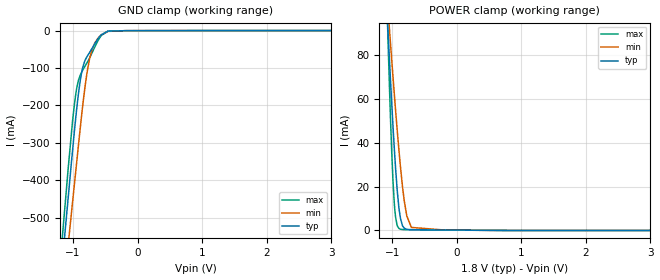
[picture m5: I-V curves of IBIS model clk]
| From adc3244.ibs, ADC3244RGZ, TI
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|   clk Model
[Model]   clk
Model_type   Input
Vinl = 0.4
Vinh = 1.2
|   typ   min   max
|   (nom PVT)   (fast PVT)   (slow PVT)
C_comp   2.914e-12   2.780e-12   2.974e-12
| Where nom  PVT is Nominal Process, 1.8V, 27C
|   Fast PVT is Strong Process,  1.9V, -40C
|   Slow PVT is Weak Process,   1.7V, 125C
[Voltage Range]   1.8   1.7   1.9
|Junction Temperature
[Temperature Range]   27   125   -40
[Power Clamp Reference]   1.8   1.7   1.9
[GND Clamp Reference]   0   0   0
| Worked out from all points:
|   POWER clamp passes 1 mA (typ) near -0.81 V on its own axis
[GND Clamp]
|   Voltage   I(typ)   I(min)   I(max)
-1.8V     -1.823A    -1.811A    -1.849A
-1.373V   -1.008A    -1.077A    -972.9mA
-1.074V   -444.1mA   -570.2mA   -366.1mA
-1.012V   -327.7mA   -465.4mA   -248.9mA
-956.4mV  -230mA     -373.3mA   -167.9mA
-863.3mV  -108.7mA   -220.2mA   -110.2mA
-811.8mV  -78.73mA   -146.5mA   -94.26mA
-746mV    -59.27mA   -76.76mA   -74.01mA
-661mV    -34.7mA    -32.49mA   -43.06mA
-560.7mV  -11.1mA    -11.08mA   -12.92mA
-180mV    -226.2uA   -175.6uA   -343.3uA
3.6V      0A         0A         0A
[POWER Clamp]
|   Voltage   I(typ)   I(min)   I(max)
-1.8V     580mA      428.2mA    963.1mA
-1.074V   95.87mA    104.5mA    95.31mA
-1.042V   76.87mA    91.28mA    64.09mA
-1.008V   57.76mA    77.61mA    35.52mA
-986.8mV  46.73mA    69.43mA    21.59mA
-948.6mV  28.52mA    54.96mA    6.132mA
-895.6mV  10.07mA    36.33mA    928.7uA
-873mV    5.522mA    29.12mA    573.8uA
-813.6mV  1.03mA     13.42mA    386.7uA
-774.9mV  497.9uA    6.66mA     368.5uA
-703.5mV  322.9uA    1.394mA    349.2uA
3.6V      0A         0A         0A
